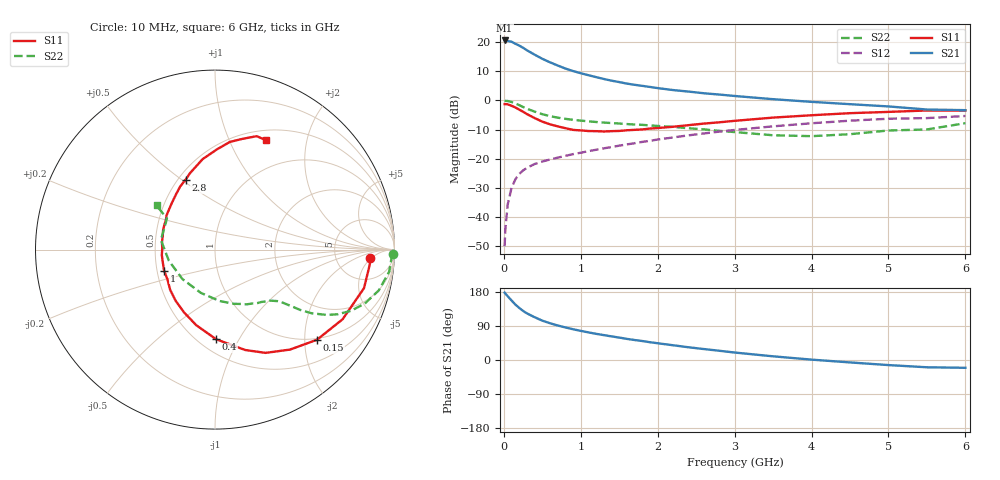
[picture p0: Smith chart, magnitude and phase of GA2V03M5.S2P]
! Infineon Technologies  Discrete & RF Semiconductors
! BF775
! Si NPN RF Bipolar Junction Transistor in SOT23
! VCE = 2 V  IC = 3.5 mA
! Common Emitter S-Parameters:  May  1996
# GHz  S  MA  R  50
!  f  S11  S21  S12  S22
! GHz  MAG  ANG  MAG  ANG  MAG  ANG  MAG  ANG
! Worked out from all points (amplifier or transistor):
!   36 points, 10 MHz to 6 GHz, reference 50 ohm
!   highest |S21| = 20.5 dB at 10 MHz (marker M1)
!   |S21| within 3 dB of that: start of sweep to 278.9 MHz
!   unconditionally stable (mu >= 1): 891.8 MHz to 4.144 GHz; 5.223 GHz to 5.958 GHz
!   at 250 MHz: K = 0.40, MSG = 21.0 dB, |S12| = -24.0 dB
!   at 1.4 GHz: K = 1.15, MAG = 9.0 dB, |S12| = -16.0 dB
!   at 6 GHz: K = 1.00, MSG = 1.0 dB, |S12| = -5.3 dB
!   S11 on the Smith chart (normalised r, x): 10 MHz: 12, -5; 150 MHz: 0.97, -2.29; 400 MHz: 0.61, -0.81; 1 GHz: 0.55, -0.14; 2.8 GHz: 0.55, +0.52; 6 GHz: 0.62, +1.38
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0.01  0.8663 -3.1  10.64 177.8  0.0032 88.4  0.9935 -1.4
0.02  0.8663 -5.6  10.5 175.1  0.0063 88.2  0.9843 -2.9
0.05  0.8575 -14.5  10.43 168.3  0.0165 81.6  0.978 -7.3
0.1  0.8101 -28.6  10.13 157.1  0.0318 74.8  0.9403 -14.0
0.15  0.7583 -41.5  9.337 146.3  0.0447 67.8  0.8873 -19.8
0.2  0.6965 -53.1  8.705 137.5  0.0552 63.4  0.8312 -24.2
0.25  0.6408 -63.9  7.978 129.5  0.0633 58.8  0.7726 -27.8
0.3  0.5846 -73.2  7.229 123.1  0.0702 56.4  0.7214 -30.3
0.4  0.4994 -89.3  6.084 112.9  0.0815 52.2  0.6442 -33.4
0.5  0.4337 -104.0  5.162 103.9  0.09 50.7  0.5822 -35.3
0.6  0.3905 -116.1  4.497 97.0  0.0975 49.9  0.538 -36.3
0.7  0.3597 -127.6  3.964 91.1  0.1049 49.9  0.5076 -37.2
0.8  0.3353 -138.2  3.518 85.9  0.1125 49.7  0.4843 -37.9
1  0.307 -157.6  2.925 76.8  0.1274 50.2  0.4515 -39.5
1.1  0.2994 -166.2  2.702 72.9  0.1355 50.5  0.4384 -40.7
1.6  0.3089 159.3  1.941 55.7  0.1768 50.7  0.3942 -47.5
2.2  0.3542 132.7  1.506 38.9  0.2326 48.3  0.3528 -59.8
2.8  0.4223 112.9  1.262 24.4  0.2925 43.4  0.3016 -77.4
3.5  0.5086 97.8  1.051 9.7  0.3603 35.6  0.2535 -108.3
4.5  0.6058 82.1  0.863 -6.4  0.4505 22.7  0.2644 -166.4
5.5  0.6734 69.8  0.699 -19.2  0.4987 7.9  0.3186 147.2
6  0.6723 64.9  0.682 -20.6  0.5418 3.8  0.4083 142.9
